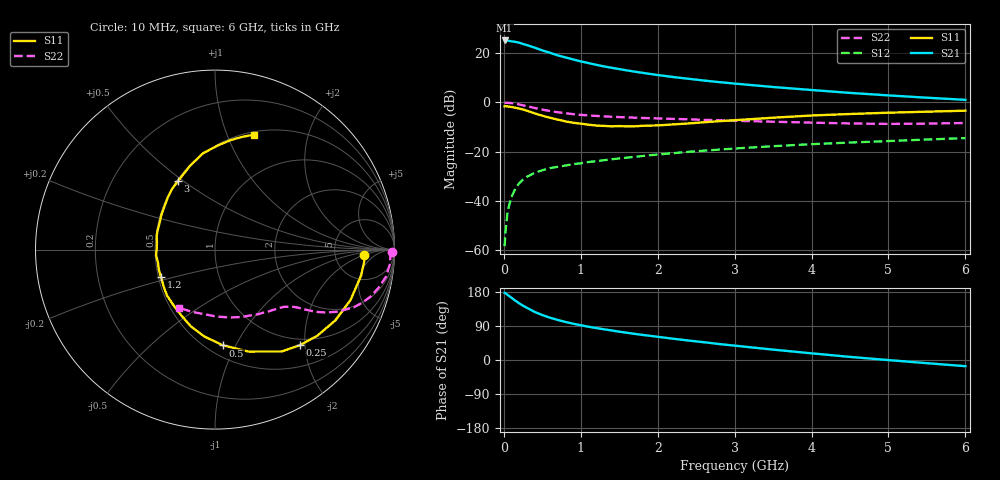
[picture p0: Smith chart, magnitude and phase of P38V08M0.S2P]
! SIEMENS Small Signal Semiconductors
! BFP181
! Si NPN RF Bipolar Junction Transistor in SOT143
! VCE = 8 V  IC = 8 mA
! Common Emitter S-Parameters:  March  1996
# GHz  S  MA  R  50
!  f  S11  S21  S12  S22
! GHz  MAG  ANG  MAG  ANG  MAG  ANG  MAG  ANG
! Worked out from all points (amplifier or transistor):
!   36 points, 10 MHz to 6 GHz, reference 50 ohm
!   highest |S21| = 25.1 dB at 10 MHz (marker M1)
!   |S21| within 3 dB of that: start of sweep to 407 MHz
!   unconditionally stable (mu >= 1): 1.529 GHz to end of sweep
!   at 250 MHz: K = 0.27, MSG = 27.5 dB, |S12| = -31.3 dB
!   at 1.4 GHz: K = 0.98, MSG = 18.6 dB, |S12| = -23.2 dB
!   at 6 GHz: K = 1.04, MAG = 6.6 dB, |S12| = -14.5 dB
!   S11 on the Smith chart (normalised r, x): 10 MHz: 10, -2; 250 MHz: 0.88, -1.90; 500 MHz: 0.60, -0.89; 1.2 GHz: 0.52, -0.18; 3 GHz: 0.51, +0.47; 6 GHz: 0.53, +1.25
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0.01  0.8307 -2.1  18.07 177.4  0.0012 84.3  0.9845 -0.7
0.02  0.8347 -4.2  18.05 176.5  0.0022 88.0  0.9777 -1.7
0.05  0.8268 -10.1  17.95 171.7  0.0063 88.7  0.9781 -4.6
0.15  0.7778 -30.5  16.91 156.5  0.0178 73.3  0.9366 -13.0
0.2  0.7449 -40.1  16.27 149.5  0.0228 69.9  0.9057 -16.8
0.25  0.7128 -48.3  15.3 143.2  0.0272 65.7  0.8704 -20.0
0.3  0.6785 -56.8  14.54 137.8  0.0307 62.5  0.8367 -22.6
0.4  0.5979 -71.8  12.91 126.9  0.0371 57.9  0.769 -26.7
0.5  0.5359 -85.1  11.34 118.6  0.0418 53.1  0.7118 -29.5
0.6  0.4871 -97.2  10.14 111.6  0.0461 51.0  0.6668 -31.4
0.7  0.447 -107.8  9.002 105.7  0.0491 49.4  0.6297 -32.7
0.8  0.41 -117.8  8.191 100.4  0.052 48.3  0.6013 -33.7
0.9  0.3851 -127.5  7.45 95.9  0.0556 47.4  0.5766 -34.5
1.1  0.3517 -144.6  6.277 87.8  0.0614 46.5  0.5419 -36.1
1.2  0.338 -152.8  5.793 84.4  0.0638 45.6  0.53 -36.9
1.7  0.3262 172.5  4.2 69.0  0.0782 44.9  0.4882 -41.5
2.2  0.3563 146.9  3.271 56.1  0.0929 42.4  0.461 -47.5
3  0.4333 118.6  2.406 37.9  0.1154 37.7  0.4228 -59.3
3.5  0.4876 106.5  2.049 27.4  0.1287 34.3  0.4045 -68.1
4.5  0.58 88.5  1.555 8.2  0.1527 26.5  0.3731 -88.8
5.5  0.6463 76.4  1.242 -8.4  0.176 19.9  0.37 -110.6
6  0.6765 71.2  1.125 -16.3  0.1876 16.0  0.381 -122.0
